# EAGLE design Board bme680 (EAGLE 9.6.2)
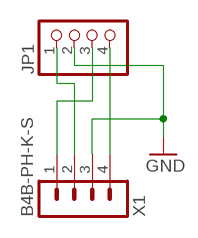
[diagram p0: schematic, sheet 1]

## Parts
JP1  PINHD-1X4  [1X04]
X1  B4B-PH-K-S  [B4B-PH-K-S]

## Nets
3.3V: JP1.1 X1.2
GND: JP1.2 X1.3
SCL: JP1.3 X1.1
SDA: JP1.4 X1.4

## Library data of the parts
JP1 = pinhead:PINHD-1X4: PIN HEADER
X1 = con-JSTPH:B4B-PH: JST PH series header 2.00mm pitch disconnectable crimp style connectors, vertical (side entry type), 4 pins

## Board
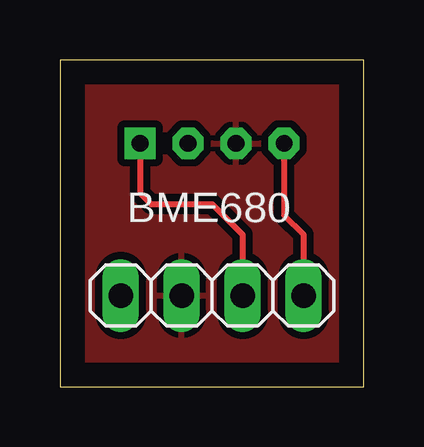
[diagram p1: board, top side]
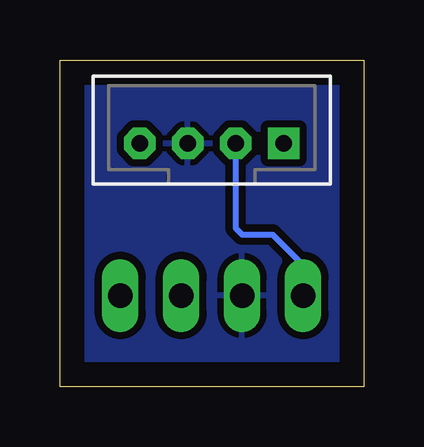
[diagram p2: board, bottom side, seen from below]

Size 12.68 x 13.64 mm. Coordinates in mm from the lower left corner, seen from the top.
Outline: 0,0 12.68,0 12.68,13.64 0,13.64 0,0
Copper layers (1*16): Top 0.035mm / dielectric 1.5mm / Bottom 0.035mm
Design rules "default": minimum track width 6mil, minimum drill 0.35mm, track to track 6mil, track to pad 6mil, pad to pad 6mil, via to via 6mil, smd to smd 6mil, copper to edge 40mil, drill to drill 6mil, minimum pad ring 10mil, minimum via ring 8mil, stop-mask expansion 4mil, vias tented up to drill 0mil, thermal gap 10mil

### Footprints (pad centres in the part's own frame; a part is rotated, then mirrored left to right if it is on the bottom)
1X04 = drill 1.016 long: 1 -3.81,0; 2 -1.27,0; 3 1.27,0; 4 3.81,0
B4B-PH-K-S = drill 0.7 pad 1.3 square: 1 3,0 | drill 0.7 pad 1.3 octagon: 2 1,0; 3 -1,0; 4 -3,0

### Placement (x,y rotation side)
JP1  6.35,3.81 0 top
X1  6.35,10.16 0 bottom

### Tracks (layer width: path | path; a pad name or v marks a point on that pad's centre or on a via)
3.3V
  Bottom 0.254: JP1.1 2.54,5.08 3.81,6.35 5.08,6.35 5.35,6.62 X1.2
GND
  pour Bottom (isolate 0.305): 0,13.97 12.7,13.97 12.7,0 0,0
  pour Top (isolate 0.305): 0,13.97 12.7,13.97 12.7,0 0,0
SCL
  Top 0.254: JP1.3 7.62,6.35 6.35,7.62 3.81,7.62 3.35,8.08 X1.1
SDA
  Top 0.254: X1.4 9.35,7.16 10.16,6.35 JP1.4

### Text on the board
tPlace: BME680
